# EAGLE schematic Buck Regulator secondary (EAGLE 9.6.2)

## Sheet 1 of 2: Datasheet
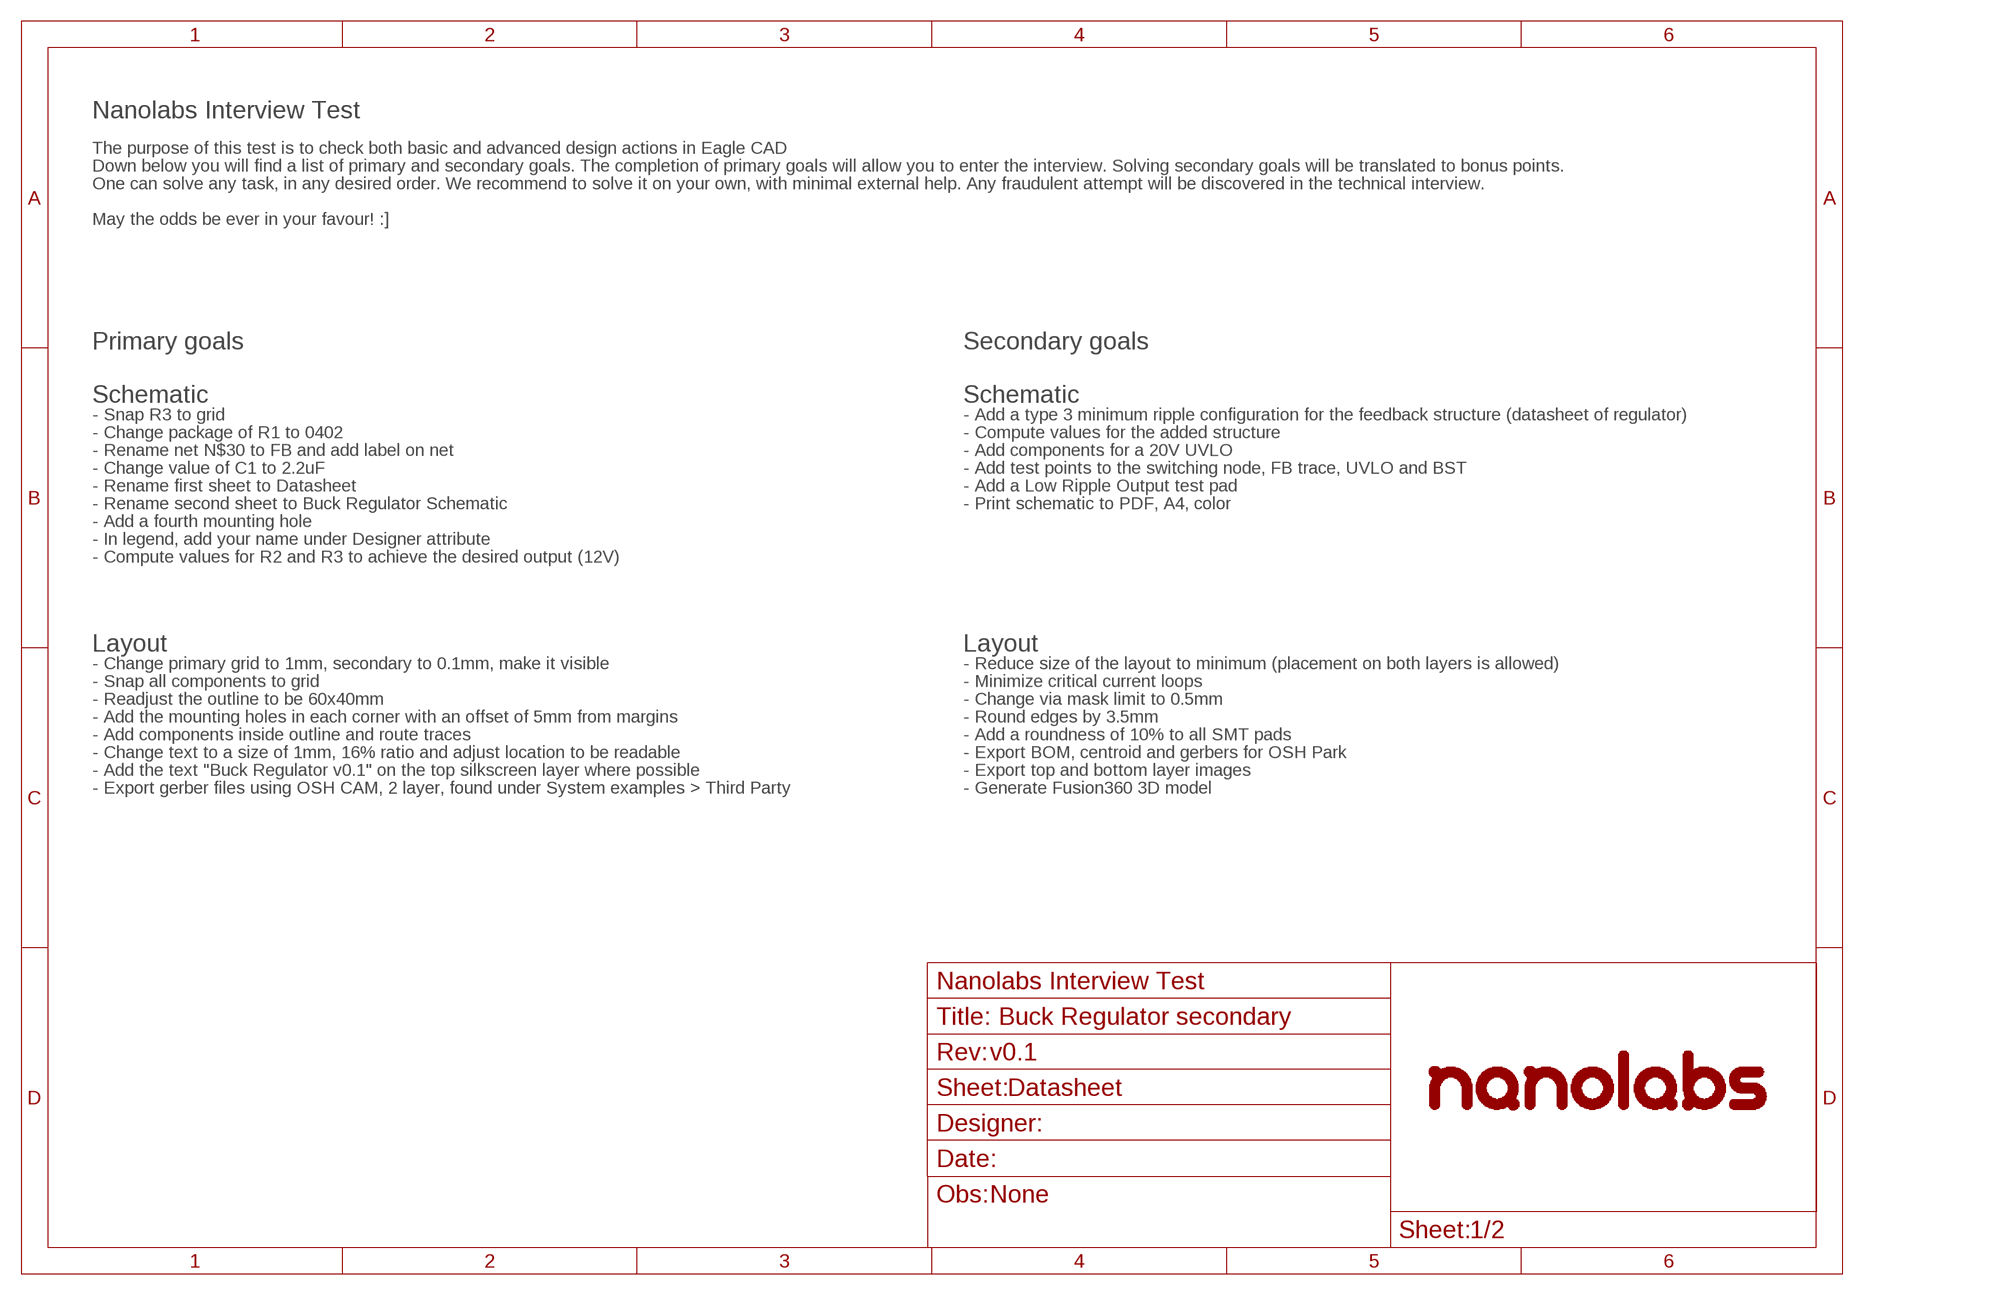
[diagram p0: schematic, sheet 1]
FRAME3 (_SCH_FRAME_A4): OBS: None; REVNUM: v0.1

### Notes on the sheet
- Nanolabs Interview Test
- The purpose of this test is to check both basic and advanced design actions in Eagle CAD
- Down below you will find a list of primary and secondary goals. The completion of primary goals will allow you to enter the interview. Solving secondary goals will be translated to bonus points.
- One can solve any task, in any desired order. We recommend to solve it on your own, with minimal external help. Any fraudulent attempt will be discovered in the technical interview.
- May the odds be ever in your favour! :]
- Primary goals | Secondary goals
- Schematic | Schematic
- - Snap R3 to grid | - Add a type 3 minimum ripple configuration for the feedback structure (datasheet of regulator)
- - Change package of R1 to 0402 | - Compute values for the added structure
- - Rename net N$30 to FB and add label on net | - Add components for a 20V UVLO
- - Change value of C1 to 2.2uF | - Add test points to the switching node, FB trace, UVLO and BST
- - Rename first sheet to Datasheet | - Add a Low Ripple Output test pad
- - Rename second sheet to Buck Regulator Schematic | - Print schematic to PDF, A4, color
- - Add a fourth mounting hole
- - In legend, add your name under Designer attribute
- - Compute values for R2 and R3 to achieve the desired output (12V)
- Layout | Layout
- - Change primary grid to 1mm, secondary to 0.1mm, make it visible | - Reduce size of the layout to minimum (placement on both layers is allowed)
- - Snap all components to grid | - Minimize critical current loops
- - Readjust the outline to be 60x40mm | - Change via mask limit to 0.5mm
- - Add the mounting holes in each corner with an offset of 5mm from margins | - Round edges by 3.5mm
- - Add components inside outline and route traces | - Add a roundness of 10% to all SMT pads
- - Change text to a size of 1mm, 16% ratio and adjust location to be readable | - Export BOM, centroid and gerbers for OSH Park
- - Add the text "Buck Regulator v0.1" on the top silkscreen layer where possible | - Export top and bottom layer images
- - Export gerber files using OSH CAM, 2 layer, found under System examples > Third Party | - Generate Fusion360 3D model

## Sheet 2 of 2: Buck Regulator Convertor
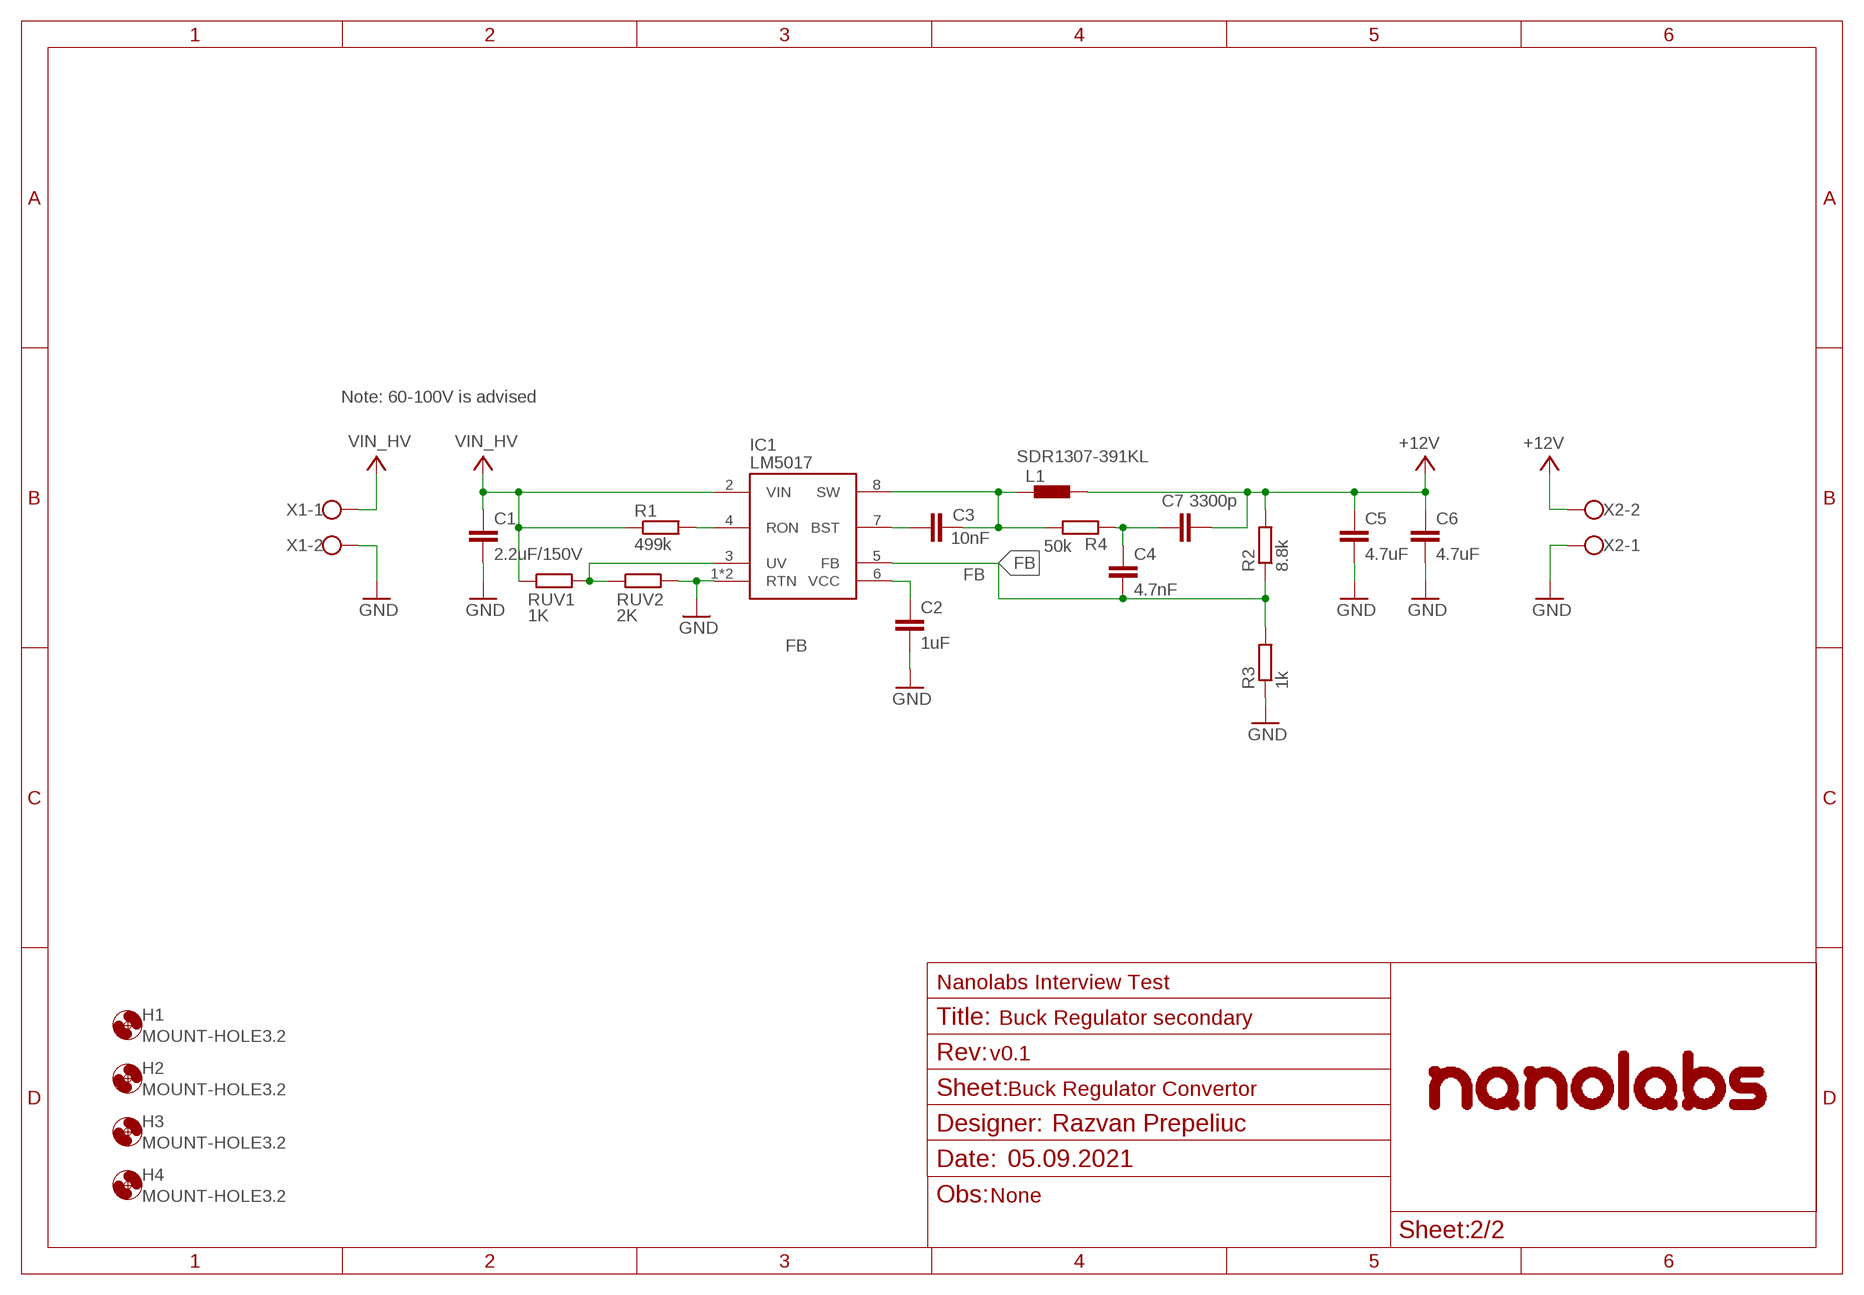
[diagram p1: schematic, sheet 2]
FRAME1 (_SCH_FRAME_A4): DNAME: 05.09.2021; OBS: None; REVNUM: v0.1

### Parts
C1  2.2uF/150V  C-EUC1812  [C1812]
C2  1uF  C-EUC0603  [C0603]
C3  10nF  C-EUC0603  [C0603]
C4  4.7nF  C-EUC0603  [C0603]
C5  4.7uF  C-EUC0603  [C0603]
C6  4.7uF  C-EUC0603  [C0603]
C7  3300p  C-EUC0603  [C0603]
H1  MOUNT-HOLE3.2  [3,2]
H2  MOUNT-HOLE3.2  [3,2]
H3  MOUNT-HOLE3.2  [3,2]
H4  MOUNT-HOLE3.2  [3,2]
IC1  LM5017  [SO-08-EP]
L1  SDR1307-391KL  [SDR1307-391KL]
R1  499k  R-EU_R0402  [R0402]
R2  8.8k  R-EU_R0603  [R0603]
R3  1k  R-EU_R0603  [R0603]
R4  50k  R-EU_R0603  [R0603]
RUV1  1K  R-EU_R0402  [R0402]
RUV2  2K  R-EU_R0402  [R0402]
X1  W237-102  [W237-102]
X2  W237-102  [W237-102]

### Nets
+12V: C5.1 C6.1 C7.2 L1.2 R2.2 X2.2
FB: C4.2 IC1.5(FB) R2.1 R3.2
GND: C1.2 C2.2 C5.2 C6.2 IC1.1(RTN) IC1.9(RTN) R3.1 RUV2.2 X1.2 X2.1
N$1: C4.1 C7.1 R4.1
N$2: IC1.3(UV) RUV1.2 RUV2.1
N$23: C2.1 IC1.6(VCC)
N$28: C3.1 IC1.7(BST)
N$29: C3.2 IC1.8(SW) L1.1 R4.2
N$31: IC1.4(RON) R1.2
VIN_HV: C1.1 IC1.2(VIN) R1.1 RUV1.1 X1.1

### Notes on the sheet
- Note: 60-100V is advised
- Razvan Prepeliuc

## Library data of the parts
C1-C7 = rcl:C-EU: CAPACITOR, European symbol; SPICEPREFIX: C
H1-H4 = _nanolabs_layout:MOUNT-HOLE: MOUNTING HOLE with drill center marker
IC1 = _nanolabs_ic:LM5017
L1 = _nanolabs_rcl:SDR1307-391KL
R1-R4 RUV1 RUV2 = rcl:R-EU_: RESISTOR, European symbol; SPICEPREFIX: R
X1 X2 = con-wago-500:W237-102: WAGO SCREW CLAMP; MPN: 237-102; OC_FARNELL: unknown; OC_NEWARK: 70K9898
